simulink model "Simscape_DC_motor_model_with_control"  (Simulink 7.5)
settings: Solver=ode45  StartTime=0.0  StopTime=20  RelTol=1e-3
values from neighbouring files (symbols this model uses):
  K = 12/4000    (= 0.003)    [INITIAL_PARAM.m]
  k2 = 12/4000    (= 0.003)    [INITIAL_PARAM.m]
  R = 10    [INITIAL_PARAM.m]
libraries: fl_lib x10, nesl_utility x4, simulink x1

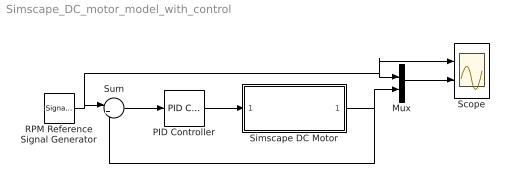
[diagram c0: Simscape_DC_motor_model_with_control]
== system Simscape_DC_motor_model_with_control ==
  Mux : Mux  Inputs=2
  PID Controller : simulink/Continuous/PID Controller  DialogController=pidpack.PIDConfig.pidDDGCreate  DialogControllerArgs=DataTag0  SystemSampleTime=-1  Controller=PID  TimeDomain=Discrete-time  SampleTime=0.01  IntegratorMethod=Forward Euler  FilterMethod=Forward Euler  Form=Parallel  P=0.263336600419252  I=3.97797577428241  D=0  N=100  InitialConditionSource=internal  InitialConditionForIntegrator=0  InitialConditionForFilter=0  ExternalReset=none  LimitOutput=off  UpperSaturationLimit=inf  LowerSaturationLimit=-inf  LinearizeAsGain=off  AntiWindupMode=none  Kb=1  TrackingMode=off  Kt=1  PParamMin=[]  PParamMax=[]  IParamMin=[]  IParamMax=[]  DParamMin=[]  DParamMax=[]  NParamMin=[]  NParamMax=[]  KbParamMin=[]  KbParamMax=[]  KtParamMin=[]  KtParamMax=[]  POutMin=[]  POutMax=[]  IOutMin=[]  IOutMax=[]  DOutMin=[]  DOutMax=[]  NOutMin=[]  NOutMax=[]  KbOutMin=[]  KbOutMax=[]  KtOutMin=[]  KtOutMax=[]  IntegratorOutMin=[]  IntegratorOutMax=[]  FilterOutMin=[]  FilterOutMax=[]  SumOutMin=[]  SumOutMax=[]  SumI1OutMin=[]  SumI1OutMax=[]  SumI2OutMin=[]  SumI2OutMax=[]  SumI3OutMin=[]  SumI3OutMax=[]  SumDOutMin=[]  SumDOutMax=[]  SaturationOutMin=[]  SaturationOutMax=[]  IntegratorContinuousStateAttributes=''  IntegratorStateMustResolveToSignalObject=off  IntegratorRTWStateStorageClass=Auto  FilterContinuousStateAttributes=''  FilterStateMustResolveToSignalObject=off  FilterRTWStateStorageClass=Auto
  RPM Reference Signal Generator : SignalGenerator  WaveForm=square  Amplitude=2700  Frequency=1/10
  Scope : Scope  NumInputPorts=2
  Simscape DC Motor : Subsystem
  Sum : Sum  Inputs=|+-  OutDataType=fixdt(1, 16)  OutScaling=2^0
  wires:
  RPM Reference Signal Generator/1 -> Sum/1, Mux/1, Scope/1
  Sum/1 -> PID Controller/1
  PID Controller/1 -> Simscape DC Motor/1(Voltage)
  Simscape DC Motor/1(Speed) -> Mux/2, Sum/2
  Mux/1 -> Scope/2

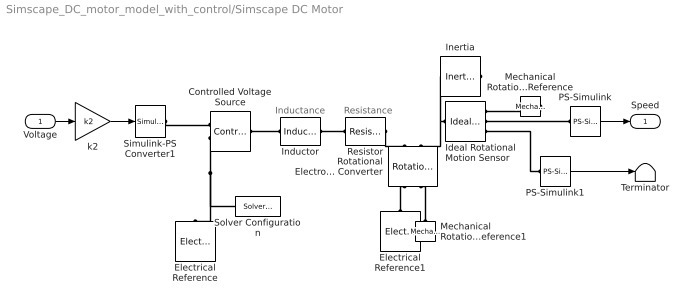
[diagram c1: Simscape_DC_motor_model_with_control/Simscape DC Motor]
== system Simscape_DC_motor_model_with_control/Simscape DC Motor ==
  note: Resistance
  note: Inductance
  Voltage : Inport  OutDataType=fixdt(1, 16)  OutScaling=2^0
  Controlled Voltage Source : fl_lib/Electrical/Electrical Sources/Controlled Voltage Source  DialogController=NetworkEngine.DynNeDlgSource  SystemSampleTime=-1  i_Log=off  v_Log=off  LocalVarNames=|i|v  LocalVarDescs=|i|v  LocalVarLogging=[0 0]
  Electrical Reference : fl_lib/Electrical/Electrical Elements/Electrical Reference  DialogController=NetworkEngine.DynNeDlgSource  SystemSampleTime=-1  i_Log=off  LocalVarNames=|i  LocalVarDescs=|i  LocalVarLogging=0
  Electrical Reference1 : fl_lib/Electrical/Electrical Elements/Electrical Reference  DialogController=NetworkEngine.DynNeDlgSource  SystemSampleTime=-1  i_Log=off  LocalVarNames=|i  LocalVarDescs=|i  LocalVarLogging=0
  Ideal Rotational Motion Sensor : fl_lib/Mechanical/Mechanical Sensors/Ideal Rotational Motion Sensor  DialogController=NetworkEngine.DynNeDlgSource  SystemSampleTime=-1  offset=0 deg  w_Log=off  t_Log=off  phi_Log=off  LocalVarNames=|w|t|phi  LocalVarDescs=|w|t|phi  LocalVarLogging=[]
  Inductor : fl_lib/Electrical/Electrical Elements/Inductor  DialogController=NetworkEngine.DynNeDlgSource  SystemSampleTime=-1  l=L mH  i0=0 A  r=0 Ohm  g=1e-9 1/Ohm  i_Log=off  v_Log=off  i_L_Log=off  LocalVarNames=|i|v|i_L  LocalVarDescs=|i|v|Internal variable for current through inductor term  LocalVarLogging=[0 0 0]
  Inertia : fl_lib/Mechanical/Rotational Elements/Inertia  DialogController=NetworkEngine.DynNeDlgSource  SystemSampleTime=-1  inertia=I kg*m^2  initial_velocity=0 rad/s  t_Log=off  LocalVarNames=|t  LocalVarDescs=|t  LocalVarLogging=0
  Mechanical Rotational Reference : fl_lib/Mechanical/Rotational Elements/Mechanical Rotational Reference  DialogController=NetworkEngine.DynNeDlgSource  SystemSampleTime=-1  t_Log=off  LocalVarNames=|t  LocalVarDescs=|t  LocalVarLogging=[]
  Mechanical Rotational Reference1 : fl_lib/Mechanical/Rotational Elements/Mechanical Rotational Reference  DialogController=NetworkEngine.DynNeDlgSource  SystemSampleTime=-1  t_Log=off  LocalVarNames=|t  LocalVarDescs=|t  LocalVarLogging=[]
  PS-Simulink : nesl_utility/PS-Simulink Converter  DialogController=NetworkEngine.DynNeUtilDlgSource  SystemSampleTime=-1  PhysicalDomain=network_engine_domain  LeftPortType=input  RightPortType=output  SubClassName=ps_output  Unit=rpm  AffineConversion=off
  PS-Simulink1 : nesl_utility/PS-Simulink Converter  DialogController=NetworkEngine.DynNeUtilDlgSource  SystemSampleTime=-1  PhysicalDomain=network_engine_domain  LeftPortType=input  RightPortType=output  SubClassName=ps_output  Unit=1  AffineConversion=off
  Resistor : fl_lib/Electrical/Electrical Elements/Resistor  DialogController=NetworkEngine.DynNeDlgSource  SystemSampleTime=-1  R=R Ohm  i_Log=off  v_Log=off  LocalVarNames=|i|v  LocalVarDescs=|i|v  LocalVarLogging=[0 0]
  Rotational Electromechanical Converter : fl_lib/Electrical/Electrical Elements/Rotational Electromechanical Converter  DialogController=NetworkEngine.DynNeDlgSource  SystemSampleTime=-1  K=K V/rpm  i_Log=off  v_Log=off  t_Log=off  w_Log=off  LocalVarNames=|i|v|t|w  LocalVarDescs=|i|v|t|w  LocalVarLogging=[0 0 0 0]
  Simulink-PS Converter1 : nesl_utility/Simulink-PS Converter  DialogController=NetworkEngine.DynNeUtilDlgSource  SystemSampleTime=-1  PhysicalDomain=network_engine_domain  LeftPortType=input  RightPortType=output  SubClassName=ps_input  Unit=V  AffineConversion=off  InputFilterTimeConstant=.001  UdotUserProvided=0
  Solver Configuration : nesl_utility/Solver Configuration  DialogController=NetworkEngine.DynNeUtilDlgSource  SystemSampleTime=-1  PhysicalDomain=network_engine_domain  LeftPortType=input  RightPortType=generic  SubClassName=solver  Accelerate=off  Profile=off  ResidualTolerance=1e-9  MaxNonlinIter=3  MaxModeIter=2  DoFixedCost=off  UseLocalSampling=off  DoDC=off  LinearAlgebra=Sparse  LocalSolverSampleTime=.001  LocalSolverChoice=NE_BACKWARD_EULER_ADVANCER  UseLocalSolver=off
  Terminator : Terminator
  k2 : Gain  Gain=k2  ParameterDataType=fixdt(1, 16)  ParameterScaling=2^0  OutDataType=fixdt(1, 16)  OutScaling=2^0
  Speed : Outport  OutDataType=fixdt(1, 16)  OutScaling=2^0
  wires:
  Voltage/1 -> k2/1
  PS-Simulink/1 -> Speed/1
  k2/1 -> Simulink-PS Converter1/1
  PS-Simulink1/1 -> Terminator/1
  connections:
  Controlled Voltage Source/LConn1 -- Inductor/LConn1
  Simulink-PS Converter1/RConn1 -- Controlled Voltage Source/RConn1
  Controlled Voltage Source/RConn2 -- Solver Configuration/RConn1 -- Electrical Reference/LConn1
  Electrical Reference1/LConn1 -- Rotational Electromechanical Converter/RConn1
  Ideal Rotational Motion Sensor/LConn1 -- Inertia/LConn1 -- Rotational Electromechanical Converter/LConn2
  Mechanical Rotational Reference/LConn1 -- Ideal Rotational Motion Sensor/RConn1
  PS-Simulink/LConn1 -- Ideal Rotational Motion Sensor/RConn2
  PS-Simulink1/LConn1 -- Ideal Rotational Motion Sensor/RConn3
  Inductor/RConn1 -- Resistor/LConn1
  Mechanical Rotational Reference1/LConn1 -- Rotational Electromechanical Converter/RConn2
  Resistor/RConn1 -- Rotational Electromechanical Converter/LConn1
